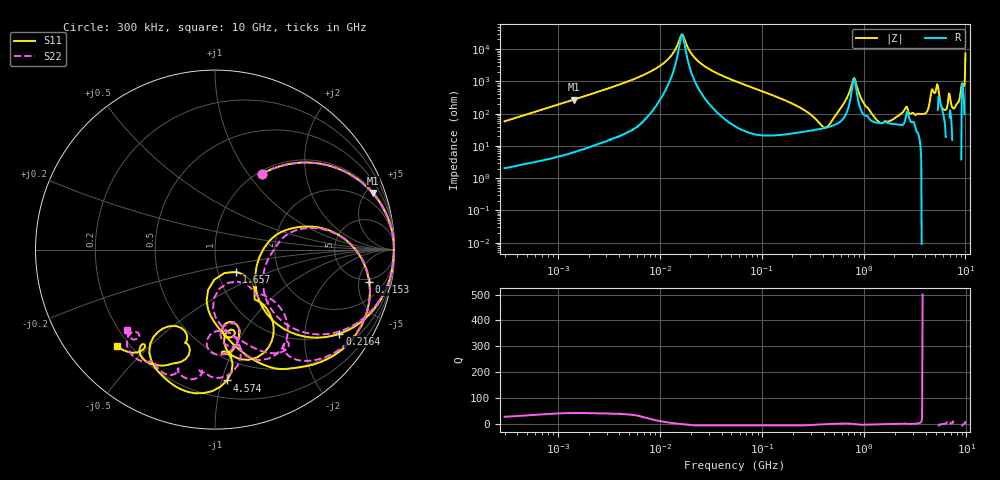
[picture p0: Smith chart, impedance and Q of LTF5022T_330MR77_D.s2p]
! S-Parameter Data Generated by TDK Corporation
! Copyright(C) 2020 TDK Corporation.
! All Rights Reserved.
! TDK P/N: LTF5022T-330MR77-D (Inductor)
! Property: L=33uH at 100kHz
! Size(LxWxT): 6.5x5x2.2mm
! Model Type: s2p (Touchstone File Format Version 1.0)
! Frequency: DC=Yes Start=0.3MHz Stop=10000MHz 802points Log-sweep
! Model Generated on Apr. 23, 2020
! Port Assignments:
!  1 ---@@@--- 2
! Applicable Conditions:
!  Temperature = 25 degC
!  DC Bias Current = 0 A
!  Small Signal Operation
! Terms and conditions regarding TDK Simulation Models
! (1)This simulation model is being provided solely for informational purposes. Please refer to the specifications of the products in terms of detailed characteristics of such products.
! (2)In no event shall TDK Corporation of any of its subsidiaries be liable for any loss or damage arising, directly or indirectly,
!  From any information contained in this simulation model, including, but not limited to loss or damages arising from any inaccuracies, omissions or errors in connection with such information.
! (3)Any and all copyrights on this simulation model are owned by TDK Corporation.
!  Duplication or redistribution of this simulation model without prior written permission from TDK Corporation is prohibited.
! (4)This simulation model is subject to any modification or change without any prior notice.
! (5)Neither TDK Corporation nor any of its subsidiaries shall make any warranty, express or implied,
!  Including but not limited to the correctness, implied warranties of merchantability and fitness for a particular purpose with respect to this simulation models.
! (6)The use of this simulation model shall be deemed to have consented to the terms and conditions hereof.
# Hz S MA R 50
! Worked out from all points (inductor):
!   801 points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, 300 kHz to 10 GHz, reference 50 ohm
!   read as one part in series: L = 30.7 uH near 318.3 kHz
!   highest Q = 42.9 at 1.44 MHz (marker M1), where L = 30.4 uH
!   self-resonance near 16.49 MHz
!   S11 on the Smith chart (normalised r, x): 300 kHz: 1.04, +1.16; 216.4 MHz: 0.95, -2.99; 715.3 MHz: 4.33, -6.87; 1.657 GHz: 1.22, -0.31; 4.574 GHz: 0.33, -1.04; 10 GHz: 0.15, -0.40
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300000  0.4955 58.3  0.8516 -29.6  0.8514 -29.7  0.4951 58.3
1439783  0.9328 19.8  0.3392 -68.9  0.3392 -68.9  0.9327 19.8
1713600  0.9502 16.8  0.2899 -71.9  0.2901 -71.9  0.9501 16.8
9671944  0.9965 1.7  0.0355 -83.8  0.03551 -83.7  0.9965 1.7
1.672204e7  0.9964 -0.6  0.003515 9.0  0.003528 8.8  0.9964 -0.5
2.441527e7  0.9961 -2.3  0.02515 79.9  0.02514 79.8  0.9961 -2.2
5.477226e7  0.9914 -7.5  0.09598 80.4  0.09599 80.4  0.9915 -7.2
2.164412e8  0.8369 -34.1  0.4434 49.0  0.4434 49.0  0.8398 -32.5
3.126428e8  0.5979 -48.6  0.627 24.5  0.627 24.5  0.6082 -45.5
4.448526e8  0.2483 -15.8  0.7146 -15.0  0.7144 -15.0  0.2952 -16.9
7.152593e8  0.878 -11.9  0.2152 -76.6  0.2151 -76.6  0.8787 -11.6
8.18524e8  0.9191 -28.4  0.07097 -11.7  0.07076 -11.6  0.9171 -27.9
1.069912e9  0.7805 -58.2  0.3479 8.5  0.3491 8.5  0.6585 -54.9
1.657186e9  0.1701 -46.9  0.4557 -25.0  0.4554 -24.6  0.1996 -67.9
1.767019e9  0.3181 -46.1  0.5867 -37.6  0.588 -37.5  0.3034 -47.1
3.72475e9  0.5366 -76.8  0.4132 -146.1  0.4166 -146.0  0.5487 -78.3
4.574322e9  0.7321 -84.8  0.09997 140.3  0.1131 139.0  0.4766 -79.2
5.284132e9  0.7389 -116.8  0.03326 44.6  0.04004 40.6  0.6854 -94.7
6.172341e9  0.483 -110.5  0.2008 -125.5  0.2026 -124.3  0.7309 -103.9
7.875699e9  0.7195 -116.4  0.132 145.7  0.1383 146.8  0.7147 -119.7
9.440974e9  0.7207 -127.3  0.01961 -111.3  0.0168 -98.8  0.6398 -131.2
1e10  0.7659 -135.2  0.001626 161.1  0.003799 -162.4  0.6646 -137.7
